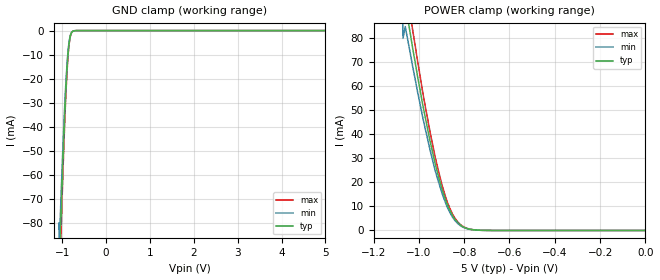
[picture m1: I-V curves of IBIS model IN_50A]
| TEXAS INSTRUMENTS INCORPORATED
| Standard Linear and Logic Group / High Volume Linear
| IBIS Model of TPD4E1U06
| Quad Channel High Speed ESD Protection Device
| This file contains package information for the following:
|  SOT 6-pin (DCK) package as [Component] TPD4E1U06_DCK
|  SOT 5-pin (DBV) package as [Component] TPD4E1U06_DBV
| This device can be powered at the following Vccs:
|  5 volt Vcc
| This file provides unique models under the [Model Selector] for each Vcc.
| For operation at a specific Vcc, select the appropriate model after each
| [Model Selector] keyword.
[IBIS Ver]   3.2
[Comment char]  |_char
[File Name]   tpd4e1u06.ibs
[File Rev]   0 | A0
[Date]   October 23, 2012
[Source]   Data created from TI-SPICE simulations at TI-SLL/HVL.
   The following is an IBIS list for the TPD4E1U06.
   Please contact sllibis@ti.com with questions and
   comments concerning SLL IBIS models.
[Notes]   Revision_History:
[Disclaimer]
| This model is designed as an aid for customers of Texas Instruments.
| TI and its licensors and suppliers make no warranties, either expressed
| or implied, with respect to this  model, including the warranties of
| merchantability or fitness for a particular purpose. The model is
| provided solely on an "as is" basis. The entire risk as to its quality
| and performance is with the customer.
[Copyright]
| (C) Copyright 2012 Texas Instruments Incorporated. All rights reserved.
| Component TPD4E1U06_DCK 6-PIN SOT
[Component]   TPD4E1U06_DCK
[Manufacturer]   Texas Instruments, Inc.
[Package]
|   typ   min   max
R_pkg   3.950e-02   1.500e-03   6.100e-02
L_pkg   4.827e-10   6.230e-12   7.072e-14
C_pkg   1.485e-13   7.072e-14   3.526e-13
[Pin]   signal_name   model_name   R_pin   L_pin   C_pin
1   D1P   IN_50A   5.614e-02   6.837e-10   1.258e-13
2   GND   GND   1.500e-03   6.250e-12   8.600e-14
3   D1N   IN_50A   5.614e-02   6.837e-10   1.253e-13
4   D2N   IN_50A   6.143e-02   7.602e-10   1.304e-13
5   NC   NC   1.500e-03   6.230e-12   7.072e-14
6   D2P   IN_50A   6.029e-02   7.558e-10   3.526e-13
| Component TPD4E1U06_DBV 5-PIN SOT
[Component]   TPD4E1U06_DBV
[Manufacturer]   Texas Instruments, Inc.
[Package]
|   typ   min   max
R_pkg   6.955e-02   3.290e-02   8.642e-02
L_pkg   1.428e-09   5.663e-10   1.646e-09
C_pkg   1.116e-13   6.352e-14   1.312e-13
[Pin]   signal_name   model_name   R_pin   L_pin   C_pin
1   D1P   IN_50A   8.640e-02   1.646e-09   1.310e-13
2   GND   GND   3.290e-03   5.663e-10   6.350e-14
3   D1N   IN_50A   8.600e-02   1.641e-09   1.310e-13
4   D2N   IN_50A   8.600e-02   1.643e-09   1.160e-13
5   D2P   IN_50A   8.600e-02   1.641e-09   1.160e-13
| Models and submodels in the file (1): IN_50A (Input)
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| Model IN
[Model]   IN_50A
Model_type  Input
Vinl=0
Vinh=5
| variable   typ   min   max
C_comp   0.64pF   0.80pF   0.96pF
[Temperature Range]   40   100   -40
| Ambient temperature   25   85   -40
[Voltage range]   5   5   5
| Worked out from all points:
|   GND clamp passes 1 mA (typ) near -0.79 V on its own axis
|   POWER clamp passes 1 mA (typ) near -0.79 V on its own axis
[GND Clamp]
| IN_50A
| Voltage   I(typ)   I(min)   I(max)
-5V       -2.25A     -2.03A     -2.48A
-1.071V   -100mA     -90mA      -110mA
-1.07V    -88.5mA    -79.7mA    -97.4mA
-1.06V    -94.03mA   -84.6mA    -103mA
-1.038V   -81.8mA    -73.6mA    -90mA
-1.027V   -75.46mA   -67.9mA    -83mA
-950mV    -36.88mA   -33.2mA    -40.6mA
-895mV    -16.3mA    -14.7mA    -17.9mA
-840mV    -4.523mA   -4.07mA    -4.98mA
-807mV    -1.625mA   -1.46mA    -1.79mA
-752mV    -224uA     -202uA     -246uA
5V        15pA       13.5pA     16.5pA
[POWER Clamp]
| IN_50A
|   Voltage   I(typ)   I(min)   I(max)
-5V       2.25A      2.03A      2.48A
-1.071V   100mA      90mA       110mA
-1.07V    88.5mA     79.7mA     97.4mA
-1.06V    94.03mA    84.6mA     103mA
-1.038V   81.8mA     73.6mA     90mA
-1.027V   75.46mA    67.9mA     83mA
-972mV    47.03mA    42.3mA     51.7mA
-917mV    23.68mA    21.3mA     26.1mA
-873mV    10.39mA    9.35mA     11.4mA
-818mV    2.309mA    2.08mA     2.54mA
-719mV    62.2uA     56uA       68.4uA
0V        0A         0A         0A
